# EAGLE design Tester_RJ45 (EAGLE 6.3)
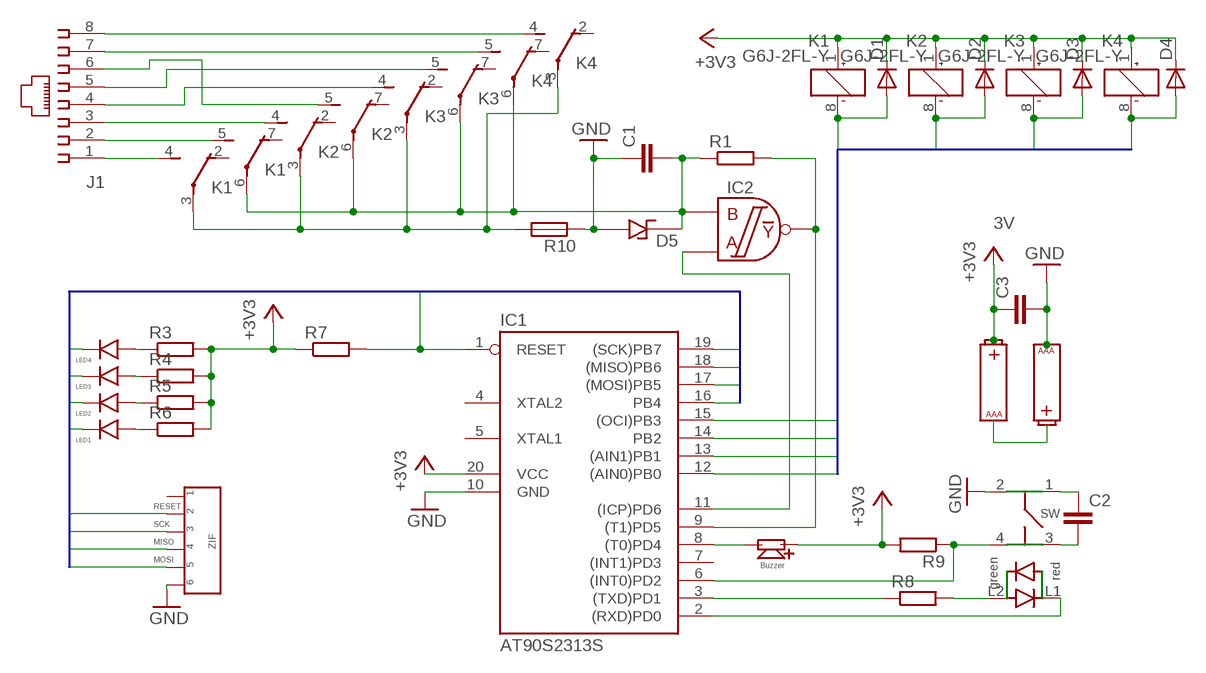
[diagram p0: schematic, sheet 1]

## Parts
BUZZER1  BMT-0905XH05  [BMT-0905XH05]
C1  C-EUC0805  [C0805]
C2  C-EUC0805  [C0805]
C3  C-EUC0805  [C0805]
D1  DIODE-MICROMELF-W  [MICROMELF-W]
D2  DIODE-MICROMELF-W  [MICROMELF-W]
D3  DIODE-MICROMELF-W  [MICROMELF-W]
D4  DIODE-MICROMELF-W  [MICROMELF-W]
D5  DIODA_TRANSILPESD5V0S1BA  [SOD323]
F1  FIBER_LED0805  [0805_FIBER]
IC1  AT90S2313S  [SO20L]
J1  555764-1  [555764-1]
K1  G6J-2FL-Y  [G6J-2FL-Y]
K2  G6J-2FL-Y  [G6J-2FL-Y]
K3  G6J-2FL-Y  [G6J-2FL-Y]
K4  G6J-2FL-Y  [G6J-2FL-Y]
R1  R-EU_R0805  [R0805]
R3  R-EU_R0805  [R0805]
R4  R-EU_R0805  [R0805]
R5  R-EU_R0805  [R0805]
R6  R-EU_R0805  [R0805]
R7  R-EU_R0805  [R0805]
R8  R-EU_R0805  [R0805]
R9  R-EU_R0805  [R0805]
R10  R-EU_R1210  [R1210]
SW1  SWITCH_PB6149L  [PB6149L__102]
U$1  AAA_BATTERY  [AAA_HOLDER]
U$2  AAA_BATTERY  [AAA_HOLDER]
U$3  MC74VHC1G132  [SOT23-5]
U$4  ZIF_CONNECTOR  [ZIF_SMT]

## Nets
2: U$1.1 U$1.2 U$2.3 U$2.4
+3V3: BUZZER1.P$1 C3.1 D1.C D2.C D3.C D4.C IC1.20(VCC) K1.1(1:+) K2.1(1:+) K3.1(1:+) K4.1(1:+) R3.2 R4.2 R5.2 R6.2 R7.1 R9.2 U$2.1 U$2.2
GND: C1.1 D5.P$1 IC1.10(GND) R10.1 SW1.2 U$4.P$6
N$1: J1.1 K1.4(2:S)
N$2: J1.2 K1.5(3:S)
N$3: J1.3 K2.4(2:S)
N$4: J1.6 K2.5(3:S)
N$5: J1.4 K3.4(2:S)
N$6: J1.5 K3.5(3:S)
N$7: J1.7 K4.5(3:S)
N$8: J1.8 K4.4(2:S)
N$9: IC1.9((T1)PD5) R1.2 U$3.P$4
N$10: C1.2 D5.P$2 K1.6(3:P) K2.6(3:P) K3.6(3:P) K4.6(3:P) R1.1 U$3.P$1
N$11: D1.A IC1.12((AIN0)PB0) K1.8(1:-)
N$12: D2.A IC1.13((AIN1)PB1) K2.8(1:-)
N$13: D3.A IC1.14(PB2) K3.8(1:-)
N$14: D4.A IC1.15((OCI)PB3) K4.8(1:-)
N$15: F1.P$7 R3.1
N$16: F1.P$5 R4.1
N$17: F1.P$3 R5.1
N$18: F1.P$1 R6.1
N$19: IC1.1(RESET) R7.2 U$4.P$2
N$20: F1.P$2 IC1.16(PB4)
N$21: F1.P$4 IC1.17((MOSI)PB5) U$4.P$5
N$22: F1.P$6 IC1.18((MISO)PB6) U$4.P$4
N$23: F1.P$8 IC1.19((SCK)PB7) U$4.P$3
N$24: IC1.3((TXD)PD1) R8.1
N$25: R8.2 SW1.L2
N$26: IC1.2((RXD)PD0) SW1.L1
N$27: IC1.6((INT0)PD2) R9.1 SW1.4
N$28: BUZZER1.P$2 IC1.8((T0)PD4)
N$29: C2.2 SW1.3
N$30: C2.1 SW1.1
N$31: IC1.11((ICP)PD6) U$3.P$2
N$34: K1.3(2:P) K2.3(2:P) K3.3(2:P) K4.3(2:P) R10.2
N$73: C3.2 U$1.3 U$1.4 ; supply symbol labelled GND
Unconnected: IC1.4(XTAL2) IC1.5(XTAL1) IC1.7((INT1)PD3) K1.2(2:O) K1.7(3:O) K2.2(2:O) K2.7(3:O) K3.2(2:O) K3.7(3:O) K4.2(2:O) K4.7(3:O) U$3.P$3 U$3.P$5 U$4.P$1

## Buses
B$1
B$2

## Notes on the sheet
- IC2
- 3V
- D5
- RESET
- SCK
- MISO
- MOSI

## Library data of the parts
BUZZER1 = BMT-0905XH05:BMT-0905XH05: Buzzer with generator 5V
C1-C3 = rcl:C-EU: CAPACITOR, European symbol
D1-D4 = diode:DIODE-: DIODE
D5 = Transil PESD5V0S1BA:DIODA_TRANSIL: Transil Diode 5V 130W
F1 = Fiber led holder 0805:FIBER_LED0805: MENTOR 1296.1004 -Fiber Led 0805 holder
IC1 = atmel:AT90S2313: MICROCONTROLLER 2 Kbytes FLASH 128 bytes SRAM 128 bytes EEPROM UART; OC_FARNELL: unknown; OC_NEWARK: unknown
J1 = con-amp:555764-1: AMP connector
K1-K4 = relay:G6J*-2?-Y: Surface-Mounting Signal Relay - G6J-Y 5.7 x 10.6 x 9 mm Source: http://www.omroncomponents.eu/ .. K125-E2-02-X.pdf; MPN: G6J-2FL-Y-TR DC4.5; OC_FARNELL: 1798618; OC_NEWARK: 04M9907
R1 R3-R10 = rcl:R-EU_: RESISTOR, European symbol
SW1 = Switch PB6149L:SWITCH_PB6149L
U$1 U$2 = AAA battery:AAA_BATTERY
U$3 = MC74VHC1G132:MC74VHC1G132: 2-Input NAND Schmitt-Trigger
U$4 = ZIF Connector:ZIF_CONNECTOR: ZIF mx52207 6 pin

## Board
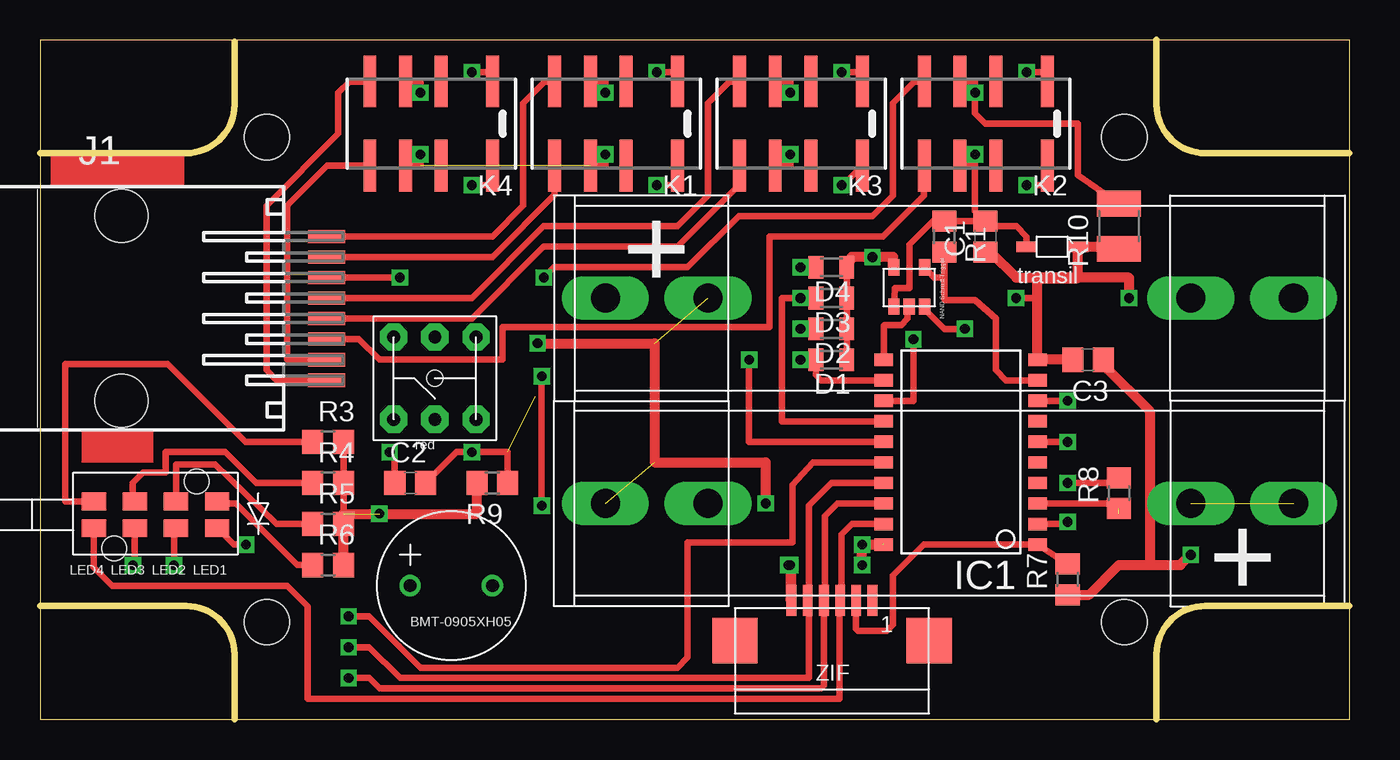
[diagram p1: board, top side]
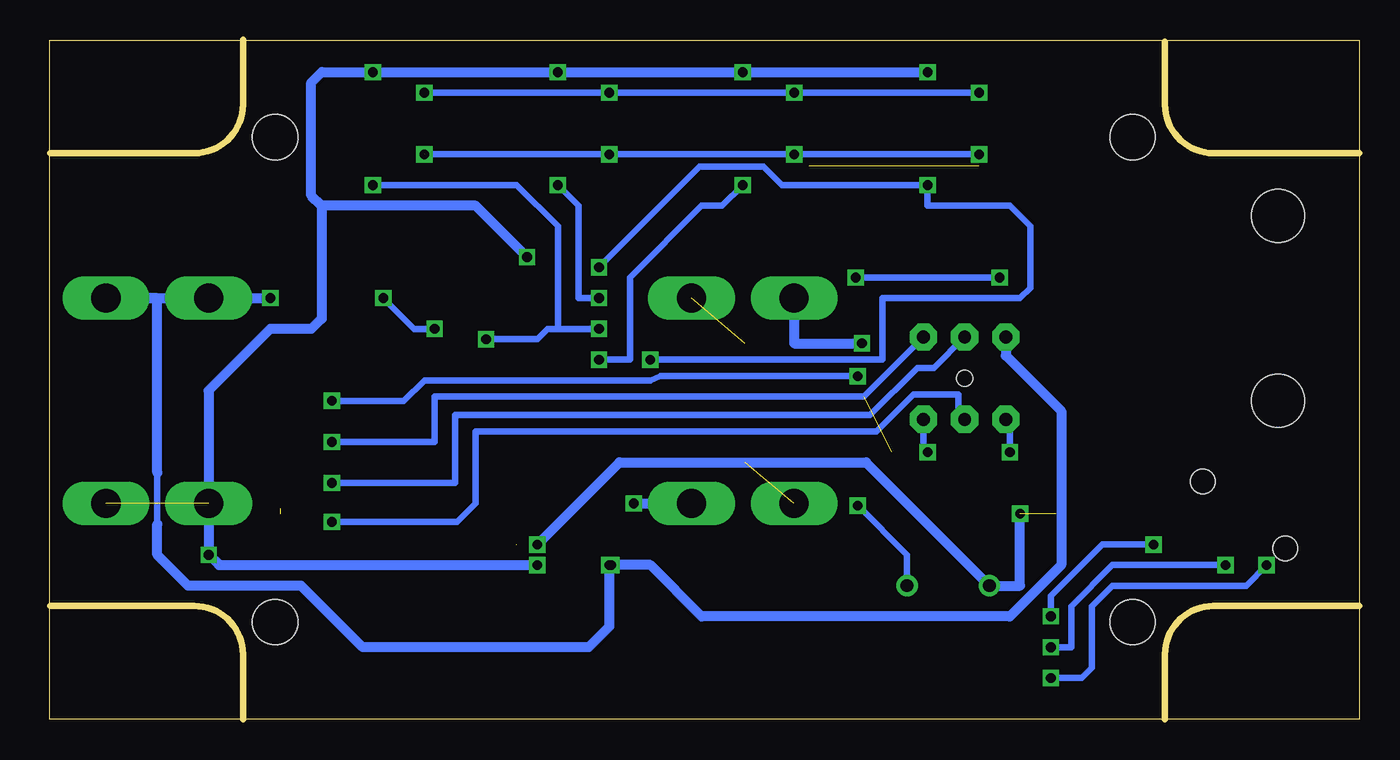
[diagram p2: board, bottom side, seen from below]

Size 80.93 x 41.97 mm. Coordinates in mm from the lower left corner, seen from the top.
Outline: 0,0 80.93,0 80.93,41.97 0,41.97 0,0
Copper layers (1*16): Top 0.035mm / dielectric 1.5mm / Bottom 0.035mm
Design rules "default": minimum track width 10mil, minimum drill 24mil, track to track 8mil, track to pad 8mil, pad to pad 8mil, via to via 8mil, smd to smd 8mil, copper to edge 40mil, drill to drill 8mil, minimum pad ring 10mil, minimum via ring 8mil, stop-mask expansion 4mil, vias tented up to drill 0mil, thermal gap 10mil
Holes 2.8 mm at 14,36 14,6 67,6 67,36
Holes 1 mm at 24.38,21.08
Milling: 12 lines

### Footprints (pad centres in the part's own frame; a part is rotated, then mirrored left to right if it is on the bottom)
BMT-0905XH05 = drill 0.8: P$1 -2.54,0; P$2 2.54,0
C0805 = smd 1.3 x 1.5: 1 -0.95,0; 2 0.95,0
MICROMELF-W = smd 0.9 x 1.4: A 0.95,0; C -0.95,0
SOD323 = smd 1.27 x 0.635: P$1 -0.635,0; P$2 2.54,0
0805_FIBER = smd 1.5 x 1.1: P$1 0,0.508; P$2 0,2.159; P$3 2.54,0.508; P$4 2.54,2.159; P$5 5.08,0.508; P$6 5.08,2.159; P$7 7.62,0.508; P$8 7.62,2.159 | hole 1.5: 1.27,-0.737; 6.35,3.404
SO20L = smd 0.762 x 1.143: 1 -5.08,-5.131; 2 -3.81,-5.131; 3 -2.54,-5.131; 4 -1.27,-5.131; 5 0,-5.131; 6 1.27,-5.131; 7 2.54,-5.131; 8 3.81,-5.131; 9 5.08,-5.131; 10 6.35,-5.131; 11 6.35,4.369; 12 5.08,4.394; 13 3.81,4.394; 14 2.54,4.394; 15 1.27,4.394; 16 0,4.394; 17 -1.27,4.394; 18 -2.54,4.394; 19 -3.81,4.394; 20 -5.08,4.394
555764-1 = smd 0.813 x 2.286: 1 -4.445,11.533; 2 -3.175,11.533; 3 -1.905,11.533; 4 -0.635,11.533; 5 0.635,11.533; 6 1.905,11.533; 7 3.175,11.533; 8 4.445,11.533 | hole 3.251: -5.715,-1.143; 5.715,-1.143
G6J-2FL-Y = smd 0.8 x 3.2: 1 -3.2,-2.6; 2 0,-2.6; 3 2.2,-2.6; 4 4.4,-2.6; 5 4.4,2.6; 6 2.2,2.6; 7 0,2.6; 8 -3.2,2.6
R0805 = smd 1.3 x 1.5: 1 -0.95,0; 2 0.95,0
R1210 = smd 1.6 x 2.7: 1 -1.4,0; 2 1.4,0
PB6149L__102 = drill 0.8 pad 1.676 octagon: 1 -2.54,2.54; 2 2.54,2.54; 3 -2.54,-2.54; 4 2.54,-2.54; L1 -2.54,0; L2 2.54,0
AAA_HOLDER = drill 1.8 long: 1 0,0; 2 6.35,0; 3 42.545,0; 4 36.195,0
SOT23-5 = smd 0.7 x 1: P$1 1.85,2.435; P$2 0.9,2.435; P$3 -0.05,2.435; P$4 -0.05,0; P$5 1.85,0
ZIF_SMT = smd 0.6 x 1.9: P$1 0,1; P$2 -1,1; P$3 -2,1; P$4 -3,1; P$5 -4,1; P$6 -5,1 | smd 2.8 x 2.8: P$7 -8.5,-1.5; P$8 3.5,-1.5

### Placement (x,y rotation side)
BUZZER1  25.4,8.26 0 top
C1  58.42,29.84 90 top
C2  22.86,14.61 0 top
C3  64.77,22.23 180 top
D1  48.9,22.23 180 top
D2  48.9,24.13 180 top
D3  48.9,26.04 180 top
D4  48.9,27.94 180 top
D5  63.5,29.21 180 top
F1  10.92,13.97 180 top
IC1  56.52,15.88 90 top
J1  6.15,25.4 270 top
K1  36.2,36.83 180 top
K2  59.05,36.83 180 top
K3  47.62,36.83 180 top
K4  24.77,36.83 180 top
R1  55.88,29.84 270 top
R3  17.78,17.14 0 top
R4  17.78,14.61 0 top
R5  17.78,12.06 0 top
R6  17.78,9.53 0 top
R7  63.5,8.64 90 top
R8  66.67,13.97 90 top
R9  27.94,14.61 180 top
R10  66.67,30.48 90 top
SW1  24.38,21.08 90 top
U$1  34.92,26.04 0 top
U$2  77.47,13.34 180 top
U$3  54.61,27.94 180 top
U$4  51.44,6.35 0 top

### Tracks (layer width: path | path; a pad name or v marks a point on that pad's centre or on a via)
2  (via drill 0.6)  (2 unrouted)
  Top 0.61: v30.73,23.24 37.97,23.24 37.97,15.88 44.83,15.88 v44.83,13.34
  Bottom 0.61: U$1.1 34.92,23.24 v30.73,23.24 | v44.83,13.34 U$2.4
+3V3  (via drill 0.6)  (4 unrouted)
  Top 0.406: R3.2 R4.2 R5.2 R6.2 | D1.C D2.C D3.C D4.C | K4.1 27.96,40.01 v26.67,40.01 | v60.96,40.01 62.23,40.01 62.23,39.43 K2.1 | v38.1,40.01 39.37,40.01 39.37,39.43 K1.1 39.4,40.01 v38.1,40.01 | v49.53,40.01 50.8,40.01 50.8,39.43 K3.1 50.83,40.01 v49.53,40.01
  Top 0.61: R6.2 18.73,12.7 26.99,12.7 R9.2 | D4.C 50.16,28.57 v51.44,28.57 52.7,28.57 52.7,27.94 | v50.8,9.53 v50.8,10.79 52.07,10.79 | C3.1 65.72,21.91 68.58,19.05 68.58,9.53 | R7.1 64.84,7.69 66.67,9.53 68.58,9.53 | 68.58,9.53 70.48,9.53 71.12,10.16
  Bottom 0.406: v26.67,40.01 v38.1,40.01 v49.53,40.01 v60.96,40.01
  Bottom 0.61: v51.44,28.57 54.61,31.75 64.14,31.75 | 64.14,31.75 64.77,32.38 64.77,39.37 64.14,40.01 v60.96,40.01 v26.67,40.01 | 20.95,12.7 20.95,8.26 BUZZER1.P$1 30.48,15.88 45.72,15.88 v50.8,10.79 | v50.8,9.53 70.48,9.53 71.12,10.16 U$2.2 71.12,20.32 67.31,24.13 64.77,24.13 64.14,24.77 64.14,31.75
GND  (via drill 0.6)
  Top 0.61: IC1.10 61.65,27.25 | 61.65,27.25 61.59,27.3 60.33,27.3 58.73,28.89 C1.1 | 61.65,27.25 64.08,27.25 64.14,27.3 | 64.14,27.3 D5.P$1 67.18,29.21 R10.1 | v67.31,26.04 67.31,27.3 64.14,27.3 | v46.35,9.53 46.35,7.43 U$4.P$6 46.44,9.45 v46.35,9.53
  Bottom 0.406: 74.3,12.06 74.3,15.24
  Bottom 0.61: SW1.2 21.84,22.48 18.41,19.05 18.41,9.53 21.59,6.35 40.64,6.35 43.81,9.53 v46.35,9.53 46.35,5.71 47.62,4.45 61.59,4.45 65.41,8.26 72.39,8.26 74.3,10.16 74.3,12.06 | 74.3,26.04 v67.31,26.04 | 74.3,15.24 74.3,26.04 | 74.3,26.04 77.47,26.04
N$1
  Top 0.406: K1.4 31.18,39.43 29.84,38.1 29.84,31.75 27.94,29.84 J1.1
N$2
  Top 0.406: K1.5 31.8,32.43 27.94,28.57 J1.2
N$3  (via drill 0.6)
  Top 0.406: K2.4 54.03,39.43 52.7,38.1 52.7,32.38 51.44,31.11 43.18,31.11 40.01,27.94 31.75,27.94 v31.11,27.3 | v22.23,27.3 J1.3
  Bottom 0.406: v31.11,27.3 v22.23,27.3
N$4
  Top 0.406: J1.6 19.68,23.5 20.95,22.23 28.57,22.23 28.57,24.26 45.09,24.26 45.09,29.84 52.07,29.84 54.61,32.38 54.61,34.19 K2.5
N$5
  Top 0.406: K3.4 42.6,39.43 41.27,38.1 41.27,32.38 39.37,30.48 31.11,30.48 26.67,26.04 J1.4
N$6
  Top 0.406: K3.5 43.23,33.06 39.37,29.21 31.11,29.21 26.67,24.77 J1.5
N$7
  Top 0.406: K4.5 17.72,34.23 15.24,31.75 15.24,22.23 J1.7
N$8
  Top 0.406: K4.4 19.11,39.43 18.41,38.73 18.41,36.2 13.97,31.75 13.97,21.59 14.61,20.95 J1.8
N$9
  Top 0.406: 55.88,27.3 55.88,25.98 55.93,25.91 57.78,25.91 59.05,24.77 59.05,21.59 59.69,20.95 IC1.9 | 55.88,27.3 R1.2 | U$3.P$4 55.24,27.3 55.88,27.3
N$10  (via drill 0.6)  (2 unrouted)
  Top 0.406: K4.6 23.5,34.23 v23.5,34.92 | K1.6 34.92,34.23 34.92,34.92 | K3.6 46.35,34.23 v46.35,34.92 | K2.6 57.78,34.23 | 57.78,34.23 57.78,34.92 | 57.78,34.23 57.78,31.43 C1.2 | C1.2 R1.1 55.18,30.8 53.72,29.34 53.72,26.67 52.83,26.67 U$3.P$1 | D5.P$2 60.96,29.84 60.33,30.48 58.73,30.48 C1.2
  Bottom 0.406: v23.5,34.92 v46.35,34.92 57.78,34.92
N$11  (via drill 0.6)
  Top 0.406: K1.8 39.37,34.23 39.37,33.02 v38.1,33.02 | v46.99,22.23 D1.A 47.95,21.27 48.26,20.95 IC1.12
  Bottom 0.406: v38.1,33.02 39.37,31.75 40.64,31.75 45.09,27.3 45.09,22.23 v46.99,22.23
N$12  (via drill 0.6)
  Top 0.406: K2.8 62.23,34.23 | 62.23,34.23 62.23,34.29 | 62.23,34.23 62.23,33.02 v60.96,33.02 | D2.A v46.99,24.13 | v53.98,23.5 53.98,19.68 IC1.13
  Bottom 0.406: v60.96,33.02 52.07,33.02 49.53,30.48 49.53,24.13 v46.99,24.13 50.16,24.13 50.8,23.5 v53.98,23.5
N$13  (via drill 0.6)
  Top 0.406: K3.8 49.62,33.02 v49.53,33.02 | v46.99,26.04 D3.A 45.85,26.04 45.85,18.41 IC1.14
  Bottom 0.406: v49.53,33.02 48.26,31.75 48.26,26.04 v46.99,26.04
N$14  (via drill 0.6)
  Top 0.406: 27.94,34.29 27.94,34.23 K4.8 27.94,34.2 27.94,33.02 v26.67,33.02 | D4.A v46.99,27.94 | IC1.15 43.81,17.14 v43.81,22.23
  Bottom 0.406: v46.99,27.94 40.77,34.16 36.83,34.16 35.69,33.02 v26.67,33.02 26.67,31.75 21.59,31.75 20.32,30.48 20.32,26.67 20.95,26.04 29.46,26.04 29.46,22.23 v43.81,22.23
N$15
  Top 0.406: F1.P$7 1.52,13.46 1.52,21.97 7.87,21.97 12.7,17.14 R3.1
N$16
  Top 0.406: F1.P$5 arc-90 5.71,13.59 5.71,14.61 6.35,15.24 7.75,15.24 7.75,16.51 11.43,16.51 13.34,14.61 R4.1
N$17
  Top 0.406: F1.P$3 8.38,15.75 10.79,15.75 14.61,12.06 R5.1
N$18
  Top 0.406: R6.1 15.88,9.53 12.06,13.34 11.05,13.34 F1.P$1
N$19
  Top 0.406: R7.2 61.71,10.73 IC1.1 54.61,10.79 52.7,8.89 52.7,5.84 52.32,5.46 50.55,5.46 50.42,5.59 50.42,7.33 U$4.P$2
N$20  (via drill 0.6)
  Top 0.406: F1.P$2 11.94,10.79 v12.7,10.79 | v19.05,6.35 20.32,6.35 23.5,3.17 39.37,3.17 40.01,3.81 40.01,10.92 46.48,10.92 46.48,14.48 47.75,15.88 IC1.16
  Bottom 0.406: v12.7,10.79 15.88,10.79 19.05,7.62 v19.05,6.35
N$21  (via drill 0.6)
  Top 0.406: F1.P$4 8.26,11.68 v8.26,9.53 | v19.05,4.45 20.32,4.45 22.23,2.54 47.5,2.54 47.5,7.16 U$4.P$5 47.5,7.41 47.5,13.21 48.9,14.61 IC1.17
  Bottom 0.406: v8.26,9.53 15.24,9.53 17.78,6.99 17.78,4.45 v19.05,4.45
N$22  (via drill 0.6)
  Top 0.406: F1.P$6 5.84,9.65 v5.71,9.53 | v19.05,2.54 20.32,2.54 20.95,1.91 48.26,1.91 48.44,2.08 U$4.P$4 48.51,7.43 48.51,12.57 49.28,13.34 IC1.18
  Bottom 0.406: v5.71,9.53 6.99,8.26 15.24,8.26 16.51,6.99 16.51,3.17 17.14,2.54 v19.05,2.54
N$23
  Top 0.406: F1.P$8 3.3,9.4 4.45,8.26 15.24,8.26 16.51,6.99 16.51,1.27 49.4,1.27 49.4,7.25 U$4.P$3 49.53,7.45 49.53,11.43 50.16,12.06 IC1.19
N$24  (1 unrouted)
  Top 0.406: IC1.3 66.67,13.34 66.67,12.7
N$25  (via drill 0.6)
  Top 0.406: R8.2 66.36,14.61 v63.5,14.61
  Bottom 0.406: v63.5,14.61 55.88,14.61 55.88,18.8 30.23,18.8 27.3,21.72 26.29,21.72 SW1.L2
N$26  (via drill 0.6)
  Top 0.406: IC1.2 63.37,12.06 v63.5,12.19
  Bottom 0.406: v63.5,12.19 55.75,12.19 54.61,13.34 54.61,17.78 29.84,17.78 27.56,20.07 24.77,20.07 24.77,18.92 SW1.L1
N$27  (via drill 0.6)  (1 unrouted)
  Top 0.406: IC1.6 v63.5,17.14 | R9.1 28.89,16.51 26.67,16.51
  Bottom 0.406: v63.5,17.14 57.15,17.14 57.15,19.94 30.61,19.94 SW1.4
N$28  (via drill 0.6)
  Top 0.406: IC1.8 v63.5,19.68 61.59,19.68 | v30.99,13.21 v30.99,21.21
  Bottom 0.406: BUZZER1.P$2 27.94,10.16 v30.99,13.21 | v30.99,21.21 43.18,21.21 43.81,20.95 57.78,20.95 59.05,19.68 v63.5,19.68
N$29  (via drill 0.6)
  Top 0.406: C2.2 25.71,16.51 v26.67,16.51
  Bottom 0.406: v26.67,16.51 26.92,16.76 SW1.3
N$30  (via drill 0.6)
  Top 0.406: v21.59,16.51 21.91,16.19 C2.1
  Bottom 0.406: SW1.1 21.59,18.29 v21.59,16.51
N$31
  Top 0.406: U$3.P$2 53.59,25.39 53.59,24.77 53.21,24.38 52.2,24.38 52.15,24.33 IC1.11
N$32  (via drill 0.6)
  other vias: 23.5,34.92
N$33  (via drill 0.6)
  other vias: 34.92,34.92
N$34  (via drill 0.6)
  Top 0.406: v34.92,38.73 34.92,39.43 K1.3 | K3.3 46.35,39.43 v46.35,38.73 | K2.3 57.78,39.43 v57.78,38.73 57.78,37.47 58.42,36.83 64.14,36.83 64.14,33.66 R10.2 | v23.5,38.73 23.5,39.37 22.57,39.37 K4.3
  Bottom 0.406: v23.5,38.73 v34.92,38.73 v46.35,38.73 v57.78,38.73
N$35  (via drill 0.6)
  other vias: 34.92,38.73
N$36  (via drill 0.6)
  other vias: 26.67,33.02
N$37  (via drill 0.6)
  other vias: 38.1,33.02
N$38  (via drill 0.6)
  other vias: 49.53,33.02
N$39  (via drill 0.6)
  other vias: 60.96,33.02
N$40  (via drill 0.6)
  other vias: 57.78,34.92
N$41  (via drill 0.6)
  other vias: 46.99,27.94
N$42  (via drill 0.6)
  other vias: 46.99,26.04
N$43  (via drill 0.6)
  other vias: 46.99,24.13
N$44  (via drill 0.6)
  other vias: 46.99,22.23
N$45  (via drill 0.6)
  other vias: 30.99,21.21
N$47  (via drill 0.6)
  other vias: 26.67,40.01
N$48  (via drill 0.6)
  other vias: 38.1,40.01
N$49  (via drill 0.6)
  other vias: 49.53,40.01
N$50  (via drill 0.6)
  other vias: 60.96,40.01
N$51  (via drill 0.6)
  other vias: 51.44,28.57
N$52  (via drill 0.6)
  other vias: 5.71,9.53
N$53  (via drill 0.6)
  other vias: 8.26,9.53
N$54  (via drill 0.6)
  other vias: 12.7,10.79
N$55  (via drill 0.6)
  other vias: 19.05,2.54
N$56  (via drill 0.6)
  other vias: 19.05,4.45
N$57  (via drill 0.6)
  other vias: 19.05,6.35
N$58  (via drill 0.6)
  other vias: 21.59,16.51
N$59  (via drill 0.6)
  other vias: 26.67,16.51
N$60  (via drill 0.6)
  other vias: 20.95,12.7
N$61  (via drill 0.6)
  other vias: 53.98,23.5
N$62  (via drill 0.6)
  other vias: 71.12,10.16
N$63  (via drill 0.6)
  other vias: 43.81,22.23
N$64  (via drill 0.6)
  other vias: 50.8,9.53
N$65  (via drill 0.6)
  other vias: 30.99,13.21
N$66  (via drill 0.6)
  other vias: 63.5,12.19
N$67  (via drill 0.6)
  other vias: 63.5,17.14
N$68  (via drill 0.6)
  other vias: 63.5,19.68
N$69  (via drill 0.6)
  other vias: 63.5,14.61
N$70  (via drill 0.6)
  other vias: 67.31,26.04
N$71  (via drill 0.6)
  other vias: 46.23,9.53
N$73  (via drill 0.6)
  Top 0.406: 54.61,25.4 55.88,24.13 v57.15,24.13 | v60.33,26.04 61.59,26.04
  Top 0.61: C3.2 61.59,22.23 61.59,26.04 61.59,27.3 67.31,27.3 v67.31,26.04
  Bottom 0.406: v57.15,24.13 58.42,24.13 v60.33,26.04
  Bottom 0.61: U$1.3 U$1.4 v67.31,26.04
N$75  (via drill 0.6)
  other vias: 30.73,23.24
N$76  (via drill 0.6)
  other vias: 44.83,13.34
(copper drawn outside any net)
  shapes: Top area x2

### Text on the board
tDocu: K4 | K1 | K3 | K2 | R1 | C1 | D5 | R10 | D4 | IC2 | J1 | sw | D3 | D2 | D1 | C3 | R3 | LED4 | LED3 | LED2 | LED1 | R9 | R4 | R8 | C2 | R5 | IC1 | R6 | R7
